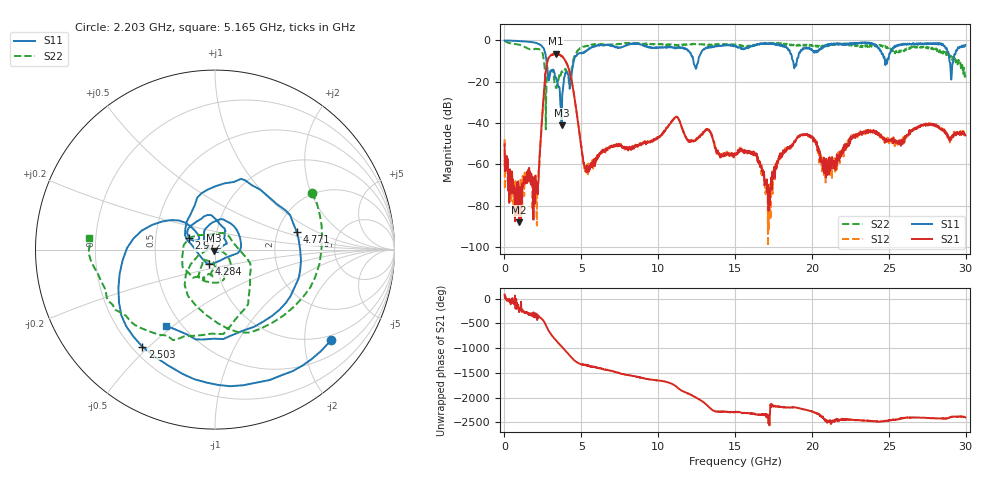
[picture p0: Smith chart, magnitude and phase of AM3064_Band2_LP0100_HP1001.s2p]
# Hz S DB R 50.0
!freq dBS11 angS11 dBS21 angS21 dBS12 angS12 dBS22 angS22
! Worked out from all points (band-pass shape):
!   1600 points, 10 MHz to 29.98 GHz, reference 50 ohm
!   highest |S21| = -6.44 dB at 3.328 GHz (marker M1); lowest = -88.0 dB at 947.2 MHz (marker M2)
!   |S21| within 3 dB of the highest: 2.823 GHz to 3.922 GHz (1.099 GHz wide, 32.6 % of centre)
!   lowest |S11| = -41.1 dB at 3.721 GHz (marker M3), VSWR 1.02, Z = 49.3 - j0.579 ohm
!   |S11| at or under -10 dB: 2.736 GHz to 4.501 GHz (1.764 GHz wide, 48.8 % of centre); 12.29 GHz to 12.6 GHz (313.7 MHz wide, 2.52 % of centre); 28.95 GHz to 29.2 GHz (255.3 MHz wide, 0.878 % of centre)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
!   |S22| runs from -43.0 to -0.2 dB; largest |S21 - S12| = 0.016
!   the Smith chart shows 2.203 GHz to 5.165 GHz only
!   S11 on the Smith chart (normalised r, x): 2.203 GHz: 0.87, -2.67; 2.503 GHz: 0.24, -0.48; 2.972 GHz: 0.74, +0.10; 4.284 GHz: 0.93, -0.15; 4.771 GHz: 2.57, +0.63; 5.165 GHz: 0.41, -0.47
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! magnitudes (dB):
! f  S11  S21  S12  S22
! 10 MHz  -0.1  -50.2  -47.9  -0.2
! 947.2 MHz  -0.3  -88.0  -82.7  -2.1
! 2.203 GHz  -1.7  -68.1  -68.8  -4.0
! 2.503 GHz  -3.4  -31.7  -31.7  -6.9
! 2.972 GHz  -16.0  -7.5  -7.4  -15.1
! 3.328 GHz  -17.9  -6.4  -6.5  -22.4
! 3.721 GHz  -41.1  -7.7  -7.5  -15.0
! 4.284 GHz  -21.1  -16.5  -16.4  -19.4
! 4.771 GHz  -6.6  -39.1  -38.8  -4.9
! 5.015 GHz  -6.4  -52.1  -51.5  -3.6
! 5.165 GHz  -5.9  -59.2  -59.7  -3.1
! 10 GHz  -3.5  -47.0  -46.8  -1.8
! 11.2 GHz  -3.6  -37.0  -36.8  -2.4
! 15 GHz  -2.7  -54.7  -53.9  -1.9
! 16.34 GHz  -2.3  -55.3  -55.6  -2.4
! 17.18 GHz  -1.8  -82.5  -92.0  -1.6
! 18.14 GHz  -3.1  -53.1  -54.6  -1.9
! 19.99 GHz  -4.5  -46.8  -46.4  -2.2
! 20.89 GHz  -2.3  -60.8  -68.7  -2.9
! 22.91 GHz  -1.3  -45.9  -45.4  -2.8
! 25 GHz  -8.5  -47.9  -49.0  -3.4
! 29.98 GHz  -2.3  -45.8  -46.4  -15.8
